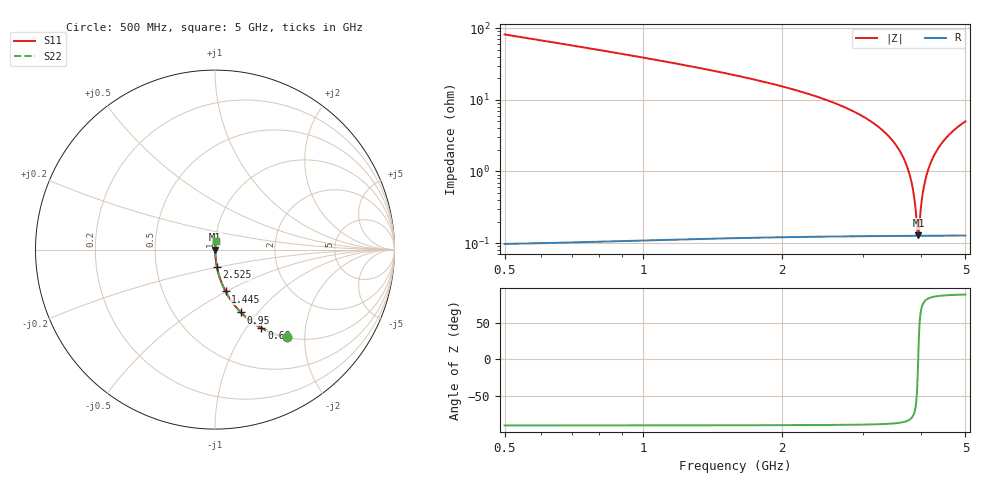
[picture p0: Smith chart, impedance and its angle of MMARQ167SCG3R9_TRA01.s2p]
! MMARQ167SCG3R9_TRA01  S-PARAMETER MODEL  ( General Type )
! Model Generated by TAIYO YUDEN Corporation (http://www.ty-top.com)
! Version 1.0
! TAIYO YUDEN Control No. 150305
! Copyright(c) 2015 TAIYO YUDEN CO.,LTD. All Rights Reserved.
! Product Description (link to TY-COMPAS)
! https://ds.yuden.co.jp/TYCOMPAS/or/detail?pn=MMARQ167SCG3R9BTRA01&u=M
! Products Name : Multilayer Ceramic Capacitors
! Characteristics :
!  Capacitance : 3.9 pF , Rated Voltage : 250V , TCC : CG / C0G
!  Case Size : 1.6 x 0.8 / 0.063 x 0.031 [mm/inch] , Thickness : 0.7 / 0.028 [mm/inch]
!  (Conditions: Temperature = 25 degC , DC Bias Current/Voltage = 0A / 0V)
! External Node Assignments :
!  1  o---| |---o  2
! GND o---------o GND
! Frequency Range : 500MHz  -  5GHz  [ 401 STEP ]
# MHz S RI R 50
! Freq[MHz].  S11 Real  S11 Imag  S21 Real  S21 Imag  S12 Real  S12 Imag  S22 Real  S22 Imag
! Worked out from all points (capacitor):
!   401 points, 500 MHz to 5 GHz, reference 50 ohm
!   read as one part in series: C = 3.85 pF near 522.5 MHz
!   lowest |Z| = 129 mohm at 3.954 GHz (marker M1)
!   series resonance near 3.949 GHz, so ESL is about 420 pH
!   S11 on the Smith chart (normalised r, x): 500 MHz: 1.00, -1.63; 680 MHz: 1.00, -1.18; 950 MHz: 1.00, -0.82; 1.445 GHz: 1.00, -0.50; 2.525 GHz: 1.00, -0.19; 5 GHz: 1.00, +0.10
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500  0.3984 -0.489  0.6016 0.489  0.6016 0.489  0.3984 -0.489
680  0.2585 -0.437  0.7415 0.437  0.7415 0.437  0.2585 -0.437
950  0.1445 -0.3503  0.8555 0.3503  0.8555 0.3503  0.1445 -0.3503
1253.75  0.0816 -0.2719  0.9184 0.2719  0.9184 0.2719  0.0816 -0.2719
1445  0.0588 -0.2329  0.9412 0.2329  0.9412 0.2329  0.0588 -0.2329
2007.5  0.0239 -0.1488  0.9761 0.1488  0.9761 0.1488  0.0239 -0.1488
2525  0.0105 -0.0956  0.9895 0.0956  0.9895 0.0956  0.0105 -0.0956
2750  0.00717 -0.0767  0.9928 0.0767  0.9928 0.0767  0.00717 -0.0767
3188.75  0.00327 -0.0449  0.9967 0.0449  0.9967 0.0449  0.00327 -0.0449
3503.75  0.00188 -0.025  0.9981 0.025  0.9981 0.025  0.00188 -0.025
3672.5  0.00149 -0.0152  0.9985 0.0152  0.9985 0.0152  0.00149 -0.0152
3785  0.00134 -0.00885  0.9987 0.00885  0.9987 0.00885  0.00134 -0.00885
3852.5  0.00129 -0.00516  0.9987 0.00516  0.9987 0.00516  0.00129 -0.00516
3886.25  0.00127 -0.00334  0.9987 0.00334  0.9987 0.00334  0.00127 -0.00334
3931.25  0.00126 -0.000934  0.9987 0.000934  0.9987 0.000934  0.00126 -0.000934
3953.75  0.00126 0.000258  0.9987 -0.000258  0.9987 -0.000258  0.00126 0.000258
4021.25  0.00128 0.00379  0.9987 -0.00379  0.9987 -0.00379  0.00128 0.00379
4077.5  0.00131 0.00669  0.9987 -0.00669  0.9987 -0.00669  0.00131 0.00669
4156.25  0.00138 0.0107  0.9986 -0.0107  0.9986 -0.0107  0.00138 0.0107
4257.5  0.00151 0.0157  0.9985 -0.0157  0.9985 -0.0157  0.00151 0.0157
4561.25  0.00218 0.0302  0.9978 -0.0302  0.9978 -0.0302  0.00218 0.0302
5000  0.00374 0.0496  0.9963 -0.0496  0.9963 -0.0496  0.00374 0.0496
